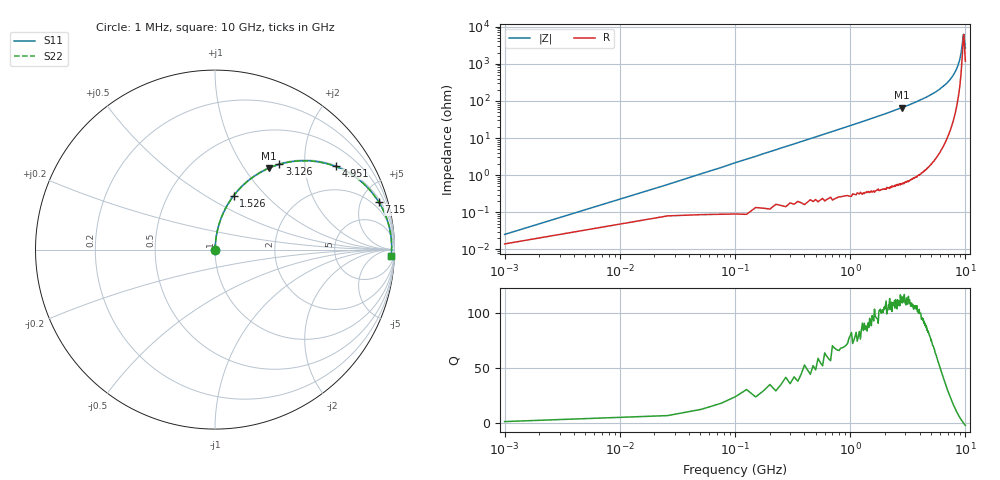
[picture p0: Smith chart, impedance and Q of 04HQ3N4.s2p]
! Coilcraft 0403HQ-3N4 Chip Inductor
! 13 February 2004
# MHZ S MA R 50
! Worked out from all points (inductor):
!   401 points, 1 MHz to 10 GHz, reference 50 ohm
!   read as one part in series: L = 3.41 nH near 50.99 MHz
!   highest Q = 112 at 2.801 GHz (marker M1), where L = 3.71 nH
!   self-resonance near 9.654 GHz
!   S11 on the Smith chart (normalised r, x): 1 MHz: 1.00, +0.00; 1.526 GHz: 1.01, +0.67; 3.126 GHz: 1.01, +1.49; 4.951 GHz: 1.03, +2.87; 7.15 GHz: 1.24, +6.76; 10 GHz: 24, -47
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1  0.000354 37.1  1 -0.0  1 -0.0  0.000354 37.1
75.992  0.016 85.8  0.999 -0.9  0.999 -0.9  0.016 85.8
100.99  0.022 86.0  0.999 -1.2  0.999 -1.2  0.022 86.0
150.985  0.032 86.0  0.998 -1.8  0.998 -1.8  0.032 86.0
275.972  0.059 85.1  0.997 -3.4  0.997 -3.4  0.059 85.1
475.952  0.101 83.1  0.993 -5.8  0.993 -5.8  0.101 83.1
725.927  0.154 80.3  0.986 -8.8  0.986 -8.8  0.154 80.3
1525.847  0.316 71.0  0.945 -18.4  0.945 -18.4  0.316 71.0
1675.832  0.345 69.2  0.935 -20.2  0.935 -20.2  0.345 69.2
2800.72  0.545 56.5  0.834 -33.0  0.834 -33.0  0.545 56.5
3125.687  0.595 52.9  0.798 -36.5  0.798 -36.5  0.595 52.9
3350.665  0.628 50.5  0.772 -38.9  0.772 -38.9  0.628 50.5
4950.505  0.816 34.6  0.568 -54.6  0.568 -54.6  0.816 34.6
5000.5  0.82 34.2  0.562 -55.1  0.562 -55.1  0.82 34.2
6675.333  0.931 19.9  0.341 -68.5  0.341 -68.5  0.931 19.9
7150.285  0.95 16.3  0.281 -71.6  0.281 -71.6  0.95 16.3
8350.165  0.978 7.9  0.139 -76.8  0.139 -76.8  0.978 7.9
9075.093  0.984 3.4  0.061 -73.0  0.061 -73.0  0.984 3.4
9275.073  0.984 2.2  0.041 -66.6  0.041 -66.6  0.984 2.2
9625.038  0.984 0.2  0.016 -10.3  0.016 -10.3  0.984 0.2
9725.028  0.984 -0.4  0.017 23.2  0.017 23.2  0.984 -0.4
10000  0.983 -1.9  0.037 61.6  0.037 61.6  0.983 -1.9
